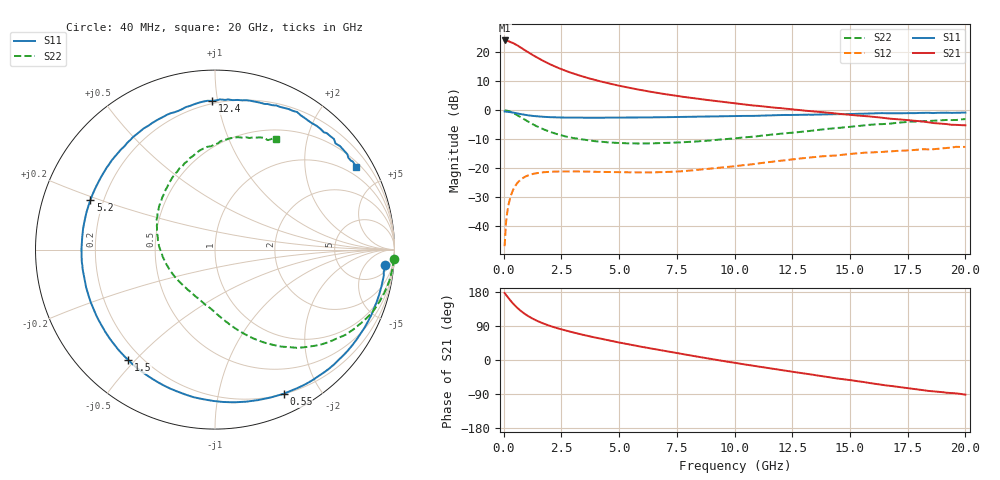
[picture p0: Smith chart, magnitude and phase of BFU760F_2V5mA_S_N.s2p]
! Filename:  P:\Prog\Test\Noise\ATS_data\Testdata_Net\BFU760\BFU760F_2W_C1_2V5mA_D.s2p
! Date/Time: Mon 06/Feb/2012 15:05:05
! BFU760_2W_C1_2V5mA
! bias mode 1: Vout= 2.0002 V, Iout= 4.9350 mA, Vin= 0.7566 V, Iin= 0.0137 mA
! Date/time Fri Mar 18 12:55:02 2011
! Device data file deembeded for feedlines and parallel
! Original file: \BFU760\BFU760_2W_C1_2V5mA_R.s2p
! Feed-files: PR003V01_101208_Feed1.s2p, PR003V01_101208_Feed2.s2p
! Parallel-file: PR003V01_101208_Par.s2p
# MHz S MA R 50
!  Freq-MHz  S11-mag  S11-arg  S21-mag  S21-arg  S12-mag  S12-arg  S22-mag  S22-arg
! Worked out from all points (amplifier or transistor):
!   167 points, 40 MHz to 20 GHz, reference 50 ohm
!   highest |S21| = 24.1 dB at 50 MHz (marker M1)
!   |S21| within 3 dB of that: start of sweep to 844.5 MHz
!   unconditionally stable (mu >= 1): 6.057 GHz to 12.72 GHz; 12.98958 GHz to 13.00592 GHz
!   at 550 MHz: K = 0.07, MSG = 24.1 dB, |S12| = -25.6 dB
!   at 4.2 GHz: K = 0.68, MSG = 15.6 dB, |S12| = -21.3 dB
!   at 20 GHz: K = 0.79, MSG = 3.7 dB, |S12| = -12.7 dB
!   lowest NFmin = 0.37 dB at 400 MHz
!   S11 on the Smith chart (normalised r, x): 40 MHz: 9, -17; 550 MHz: 0.20, -1.56; 1.5 GHz: 0.15, -0.48; 5.2 GHz: 0.15, +0.19; 12.4 GHz: 0.18, +0.96; 20 GHz: 0.65, +3.57
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40  0.9523 -5.1  16.09 176.9  0.004472 86.0  0.997 -2.9
50  0.9502 -6.9  16.11 175.6  0.00526 83.4  0.9961 -3.7
60  0.948 -7.4  15.89 174.9  0.006603 86.6  0.9962 -4.3
80  0.9506 -10.1  16.04 173.5  0.008952 84.4  0.9944 -5.8
140  0.9471 -17.6  15.85 168.7  0.01565 80.5  0.9863 -10.2
280  0.9322 -34.9  15.24 157.8  0.03031 71.3  0.9504 -20.1
420  0.9106 -51.0  14.46 148.0  0.04299 62.7  0.8965 -29.0
550  0.8897 -64.5  13.54 139.9  0.05255 55.4  0.8372 -36.5
750  0.8577 -82.8  12.1 129.1  0.06383 46.2  0.7507 -46.1
1000  0.8246 -101.4  10.43 118.2  0.07325 37.2  0.6552 -55.6
1250  0.7997 -116.2  9.053 109.3  0.07907 30.5  0.5764 -63.0
1500  0.7825 -128.1  7.946 101.9  0.08266 25.2  0.5138 -69.1
1850  0.7659 -141.4  6.707 93.3  0.08561 19.5  0.4477 -76.2
2250  0.7538 -153.1  5.648 85.2  0.08725 14.9  0.394 -83.0
3400  0.7439 -176.7  3.863 67.0  0.08746 6.6  0.3138 -99.3
5200  0.7471 158.4  2.554 43.8  0.08483 2.4  0.2704 -124.2
6800  0.7576 141.0  1.958 25.7  0.08518 3.5  0.2704 -146.6
10200  0.7972 109.7  1.291 -9.3  0.1102 5.6  0.3332 165.0
12400  0.8286 91.1  1.049 -30.0  0.1401 -0.5  0.4059 137.3
13400  0.8385 83.2  0.9577 -38.9  0.1543 -5.9  0.446 125.5
16800  0.8875 55.8  0.712 -68.6  0.1951 -26.4  0.5912 88.6
20000  0.912 30.4  0.5492 -91.4  0.2329 -49.4  0.7033 61.3
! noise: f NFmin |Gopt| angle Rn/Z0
400  0.3682  0.4372  23.53  0.0893
650  0.3809  0.4067  38.11  0.0896
1050  0.4051  0.3911  60.58  0.0876
1500  0.4384  0.4017  82.51  0.0825
1900  0.4733  0.4211  99.05  0.076
2300  0.5132  0.4436  113.7  0.0683
3000  0.595  0.4874  136.2  0.0538
3800  0.7073  0.5455  158.1  0.0389
4600  0.8395  0.6025  175.9  0.0306
6000  1.119  0.6142  198.5  0.0459
